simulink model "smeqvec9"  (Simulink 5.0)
settings: Solver=ode45  StartTime=0.0  StopTime=12  MaxStep=.05  RelTol=1e-4  AbsTol=1e-4
InitFcn:
  | smvecdef8
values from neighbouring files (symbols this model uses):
  Bm = 0.10    (= 0.1)    [IMabc2.m]    (also in imabcparam.m = 0.01; IMabcrun0.m = 0.01; IMabcrun1.m = 0.001; IMcur0.m = 1e-06)
  H = 0.60    (= 0.6)    [IMabc2.m]    (also in IMcur0.m = 0.3; imdef0vec.m = 0.3; imdef1vec.m = 0.3; imdef2vec.m = 0.3)
  Ra = .95    (= 0.95)    [altwdgs.m]    (also in Ccurverun.m = 0.018)
  V = [Vas 0 0].'    [Actac.m]    (also in acttrcalc1.m = str2num(get(h,'string')); im3d.m = eval(get(hVs,'String')); IMabc2.m = [vas vbs vcs 0 0 0]'; IMabcf0.m = [vas vbs vcs 0 0 0]')
  wo = 2*pi*freq0    [calc0.m]    (also in IMabc2.m = 376.991118431; imabcparam.m = 376.991118431; IMabcrun0.m = 376.991118431; IMabcrun1.m = 376.991118431)
undefined symbols (not defined in the file or in its folder): delta0, fa0, fk0, L_1, Lline, phif0, Rf, Rkd, Rkq, Rline, vf0
libraries: simulink x3

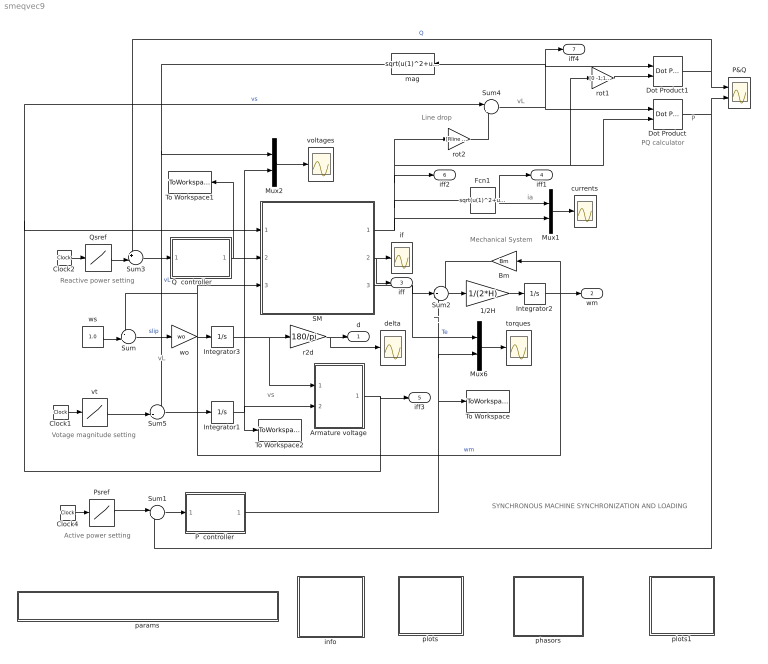
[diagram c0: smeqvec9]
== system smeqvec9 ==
  note: Tl
  note: P
  note: SYNCHRONOUS MACHINE SYNCHRONIZATION AND LOADING
  note: Reactive power setting
  note: Active power setting
  note: vs
  note: Mechanical System
  note: ia
  note: Votage magnitude setting
  note: PQ calculator
  note: vL
  note: i
  note: Line drop
  note: vL
  1/2H : Gain  Gain=1/(2*H)
  Armature voltage : Subsystem
  Bm : Gain  Orientation=left  Gain=Bm
  Clock1 : Clock
  Clock2 : Clock
  Clock4 : Clock
  Dot Product : simulink/Math Operations/Dot Product
  Dot Product1 : simulink/Math Operations/Dot Product
  Fcn1 : Fcn  Expr=sqrt(u(1)^2+u(2)^2)
  Integrator1 : Integrator  InitialCondition=V
  Integrator2 : Integrator  InitialCondition=1
  Integrator3 : Integrator  InitialCondition=delta0
  Mux1 : Mux  Inputs=2
  Mux2 : Mux  Inputs=2
  Mux6 : Mux  Inputs=2
  P  controller : Subsystem  mask{Kp=.2, Ki=1, sat=3}
      mask prompts: Kp "Proportional gain (Kp)"; Ki "Integral gain (Ki)"; sat "Saturation limit [pu]"
      mask help: Proportional-Integral Speed Controller
  P&Q : Scope  NumInputPorts=2
  Psref : Lookup  InputValues=[0 2 2.01 10]  OutputValues="[0 0  -1 -1]"
  Q  controller : Subsystem  mask{Kp=.1, Ki=.2, sat=.1}
      mask prompts: Kp "Proportional gain (Kp)"; Ki "Integral gain (Ki)"; sat "Saturation limit [pu]"
      mask help: Proportional-Integral Speed Controller
  Qsref : Lookup  InputValues=[0 5 5.01 10]  OutputValues="[0 0  -.3 -.3 ]"
  SM : Subsystem
  Sum : Sum  Inputs=-+|
  Sum1 : Sum  Inputs=|+-
  Sum2 : Sum  Inputs=-+-
  Sum3 : Sum  Inputs=+-|
  Sum4 : Sum  Inputs=|++
  Sum5 : Sum  Inputs=-+|
  To Workspace : ToWorkspace  VariableName=Tl0  SampleTime=-1  SaveFormat=StructureWithTime
  To Workspace1 : ToWorkspace  VariableName=vf0  SampleTime=-1  SaveFormat=StructureWithTime
  To Workspace2 : ToWorkspace  VariableName=vs0  SampleTime=-1  SaveFormat=Array
  currents : Scope
  delta : Scope
  if : Scope
  info : Subsystem
  mag : Fcn  Orientation=left  Expr=sqrt(u(1)^2+u(2)^2)
  params : Subsystem
  phasors : Subsystem
  plots : Subsystem
  plots1 : Subsystem
  r2d : Gain  Gain=180/pi
  rot1 : Gain  Gain=[0 -1;1 0]  Multiplication=Matrix(K*u)
  rot2 : Gain  Gain=[Rline -Lline;Lline Rline]  Multiplication=Matrix(K*u)
  torques : Scope
  voltages : Scope
  vt : Lookup  InputValues=[0 1 1.01 20 ]  OutputValues=[V V 1.0 1.0]
  wo : Gain  Gain=wo
  ws : Constant  Value=1.0
  d : Outport
  wm : Outport  Port=2
  iff : Outport  Port=3
  iff1 : Outport  Port=4
  iff3 : Outport  Port=5
  iff2 : Outport  Port=6
  iff4 : Outport  Port=7
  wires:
  1/2H/1 -> Integrator2/1
  Sum2/1 -> 1/2H/1
  Bm/1 -> Sum2/1
  SM/3(Te) -> Mux6/1, Sum2/2  "Te"
  Mux6/1 -> torques/1
  SM/1(ia) -> Mux1/2, Fcn1/1, iff2/1, rot1/1, Dot Product/2, rot2/1
  SM/2(if) -> if/1, iff/1
  Integrator2/1 -> Bm/1, wm/1, SM/3(wm), Sum/1  "wm"
  Dot Product/1 -> P&Q/2, Sum1/2
  Dot Product1/1 -> P&Q/1, Sum3/1  "Q"
  rot1/1 -> Dot Product1/2
  Fcn1/1 -> iff1/1, Mux1/1
  Mux1/1 -> currents/1
  r2d/1 -> delta/1, d/1
  Sum3/1 -> Q  controller/1(Q_er)
  Clock2/1 -> Qsref/1
  Q  controller/1(vf) -> SM/2(vf), To Workspace1/1
  Armature voltage/1(vs) -> iff3/1, SM/1(vs), Sum4/1  "vs"
  Qsref/1 -> Sum3/2
  Sum1/1 -> P  controller/1(P_er)
  Clock4/1 -> Psref/1
  P  controller/1(Tmec) -> Sum2/3, Mux6/2, To Workspace/1
  ws/1 -> Sum/2
  Sum/1 -> wo/1  "slip"
  wo/1 -> Integrator3/1
  Integrator3/1 -> Armature voltage/1(delta), r2d/1
  Psref/1 -> Sum1/1
  Clock1/1 -> vt/1
  Sum4/1 -> Dot Product/1, Dot Product1/1, iff4/1, mag/1
  rot2/1 -> Sum4/2
  vt/1 -> Sum5/2
  Sum5/1 -> Integrator1/1
  Integrator1/1 -> Armature voltage/2(Vt), Mux2/2, To Workspace2/1
  mag/1 -> Sum5/1, Mux2/1  "vL"
  Mux2/1 -> voltages/1

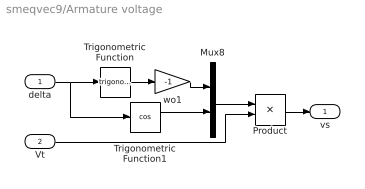
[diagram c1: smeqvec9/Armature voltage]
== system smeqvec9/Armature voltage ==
  delta : Inport
  Vt : Inport  Port=2
  Mux8 : Mux  Inputs=2
  Product : Product
  Trigonometric Function : Trigonometry
  Trigonometric Function1 : Trigonometry  Operator=cos
  wo1 : Gain  Gain=-1
  vs : Outport
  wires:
  delta/1 -> Trigonometric Function/1, Trigonometric Function1/1
  Trigonometric Function/1 -> wo1/1
  Mux8/1 -> Product/1
  wo1/1 -> Mux8/1
  Trigonometric Function1/1 -> Mux8/2
  Product/1 -> vs/1
  Vt/1 -> Product/2

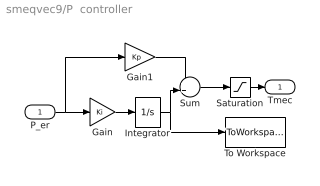
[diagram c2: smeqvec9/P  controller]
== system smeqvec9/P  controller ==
  P_er : Inport
  Gain : Gain  Gain=Ki
  Gain1 : Gain  Gain=Kp
  Integrator : Integrator  LimitOutput=on  UpperSaturationLimit=sat  LowerSaturationLimit=-sat
  Saturation : Saturate  UpperLimit=sat  LowerLimit=-sat
  Sum : Sum
  To Workspace : ToWorkspace  VariableName=xtl  SampleTime=-1  SaveFormat=Array
  Tmec : Outport  InitialOutput=0
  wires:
  Gain1/1 -> Sum/1
  Gain/1 -> Integrator/1
  P_er/1 -> Gain/1, Gain1/1
  Sum/1 -> Saturation/1
  Saturation/1 -> Tmec/1
  Integrator/1 -> Sum/2, To Workspace/1

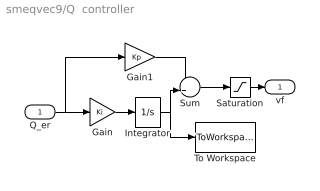
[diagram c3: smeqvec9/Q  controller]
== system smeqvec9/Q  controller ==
  Q_er : Inport
  Gain : Gain  Gain=Ki
  Gain1 : Gain  Gain=Kp
  Integrator : Integrator  InitialCondition=vf0  LimitOutput=on  UpperSaturationLimit=sat  LowerSaturationLimit=-sat
  Saturation : Saturate  UpperLimit=sat  LowerLimit=-sat
  Sum : Sum
  To Workspace : ToWorkspace  VariableName=xeq  SampleTime=-1  SaveFormat=Array
  vf : Outport  InitialOutput=0
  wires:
  Saturation/1 -> vf/1
  Sum/1 -> Saturation/1
  Q_er/1 -> Gain1/1, Gain/1
  Gain/1 -> Integrator/1
  Gain1/1 -> Sum/1
  Integrator/1 -> Sum/2, To Workspace/1

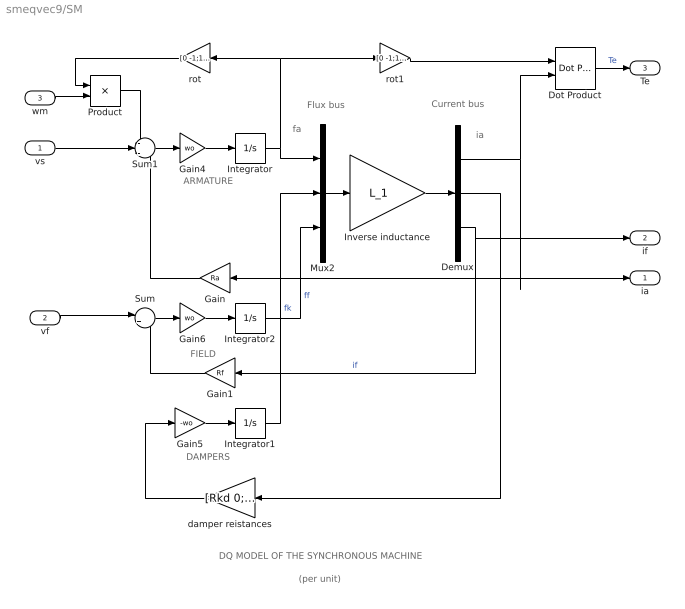
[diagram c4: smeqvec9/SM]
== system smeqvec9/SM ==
  note: DAMPERS
  note: ARMATURE
  note: fa
  note: ia
  note: FIELD
  note: DQ MODEL OF THE SYNCHRONOUS MACHINE
  note: Flux bus
  note: Current bus
  note: (per unit)
  vs : Inport
  vf : Inport  Port=2
  wm : Inport  Port=3
  Demux : Demux  Outputs=3
  Dot Product : simulink/Math Operations/Dot Product
  Gain : Gain  Orientation=left  Gain=Ra
  Gain1 : Gain  Orientation=left  Gain=Rf
  Gain4 : Gain  Gain=wo
  Gain5 : Gain  Gain=-wo
  Gain6 : Gain  Gain=wo
  Integrator : Integrator  InitialCondition=fa0
  Integrator1 : Integrator  InitialCondition=fk0
  Integrator2 : Integrator  InitialCondition=phif0
  Inverse inductance : Gain  Gain=L_1  Multiplication=Matrix(K*u)
  Mux2 : Mux  Inputs=3
  Product : Product
  Sum : Sum  Inputs=|+-
  Sum1 : Sum  Inputs=-+-
  damper reistances : Gain  Orientation=left  Gain=[Rkd 0;0 Rkq]  Multiplication=Matrix(K*u)
  rot : Gain  Orientation=left  Gain=[0 -1;1 0]  Multiplication=Matrix(K*u)
  rot1 : Gain  Gain=[0 -1;1 0]  Multiplication=Matrix(K*u)
  ia : Outport
  if : Outport  Port=2
  Te : Outport  Port=3
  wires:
  Product/1 -> Sum1/1
  rot/1 -> Product/1
  wm/1 -> Product/2
  Gain5/1 -> Integrator1/1
  damper reistances/1 -> Gain5/1
  Integrator/1 -> Mux2/1, rot/1, rot1/1
  Sum1/1 -> Gain4/1
  Gain4/1 -> Integrator/1
  vs/1 -> Sum1/2
  Gain/1 -> Sum1/3
  Gain6/1 -> Integrator2/1
  Sum/1 -> Gain6/1
  vf/1 -> Sum/1
  Gain1/1 -> Sum/2
  rot1/1 -> Dot Product/1
  Demux/1 -> Gain/1, ia/1, Dot Product/2
  Dot Product/1 -> Te/1  "Te"
  Mux2/1 -> Inverse inductance/1
  Inverse inductance/1 -> Demux/1
  Integrator1/1 -> Mux2/2  "fk"
  Integrator2/1 -> Mux2/3  "ff"
  Demux/2 -> damper reistances/1
  Demux/3 -> if/1, Gain1/1  "if"

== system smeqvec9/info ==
  note: The synchronous machine is running open circuited and close to synchronous speed when it is connected to the power system. The transients occurring during the synchronization process will depend on the initial state defined by the excitation no-load voltage Ef, the speed, and the phase (torque) angle. The machine is connected to a load bus via a line impedance. Once synchronized, the machine is loaded: the real power absorbed P (at the bus) is adjusted by controlling the input torque Tl (negatively for generator operation and positively for motor operation); the reactive power absorbed Q is adjusted by controlling the voltage vf applied to the field. The voltage at the load bus is adjusted by controlling the machine terminal voltage. To simplify the simulations, the excitation system controls and the governor drive controls are modeled by means of PI controllers. The dynamic system response is exhibited. The final steady-state conditions are described by phasors oriented along the dq axes. Once these conditions are established, the machine can then be short circuited at its terminals by double clicking the block marked .
  note: SYNCHRONOUS MACHINE
  note: SYNCHRONIZATION AND LOADING FOLLOWED BY A SHORT CIRCUIT

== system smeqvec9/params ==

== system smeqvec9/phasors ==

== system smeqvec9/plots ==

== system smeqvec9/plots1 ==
